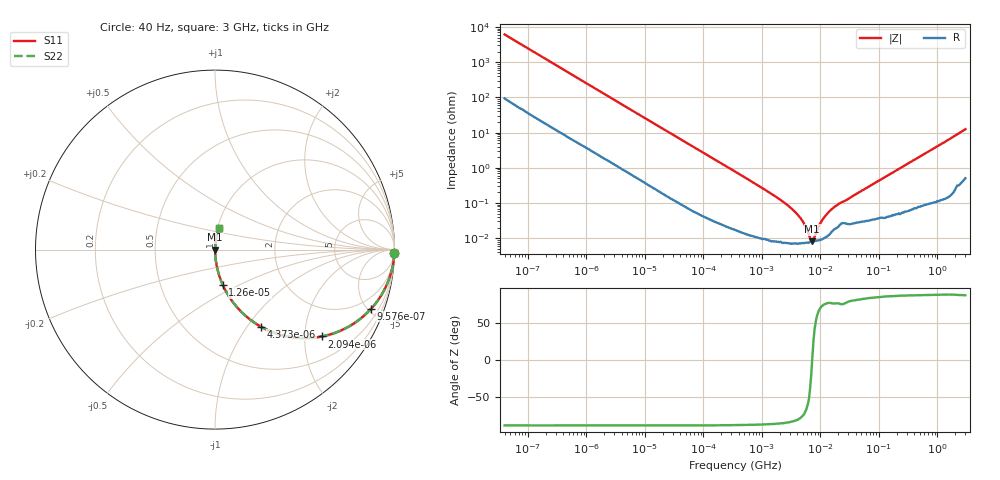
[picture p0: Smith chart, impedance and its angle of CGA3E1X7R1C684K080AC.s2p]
! S-parameter Generated by TDK Corporation
! Copyright(C) 2015 TDK Corporation.
! All Rights Reserved.
! TDK P/N: CGA3E1X7R1C684K080AC (Multilayer Ceramic Chip Capacitors)
! Property: C=680nF
! Size(LxWxT): 1.6x0.8x0.8mm, 0.063x0.031x0.031inches
! Model Type: s2p (Touchstone File Format Version 1.0)
! Frequency: DC=Yes Start=0.00004MHz Stop=3000MHz 396points Log-sweep
! Note: This model was converted from impedance.
! Model Generated on Jun. 23, 2015
! Hash(MD5):
! Port Assignments:
!  1 ---| |--- 2
! Applicable Conditions:
!  Temperature = 25 degC
!  DC Bias Voltage = 0 V
!  Small Signal Operation
! Terms and conditions regarding TDK Simulation Models
! (1)This simulation model is being provided solely for informational purposes. Please refer to the specifications of the products in terms of detailed characteristics of such products.
! (2)In no event shall TDK Corporation of any of its subsidiaries be liable for any loss or damage arising, directly or indirectly,
!  From any information contained in this simulation model, including, but not limited to loss or damages arising from any inaccuracies, omissions or errors in connection with such information.
! (3)Any and all copyrights on this simulation model are owned by TDK Corporation.
!  Duplication or redistribution of this simulation model without prior written permission from TDK Corporation is prohibited.
! (4)This simulation model is subject to any modification or change without any prior notice.
! (5)Neither TDK Corporation nor any of its subsidiaries shall make any warranty, express or implied,
!  Including but not limited to the correctness, implied warranties of merchantability and fitness for a particular purpose with respect to this simulation models.
! (6)The use of this simulation model shall be deemed to have consented to the terms and conditions hereof.
# MHz S MA R 50
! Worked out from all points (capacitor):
!   395 points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, 40 Hz to 3 GHz, reference 50 ohm
!   read as one part in series: C = 647 nF near 41.88 Hz
!   lowest |Z| = 8.17 mohm at 7.224 MHz (marker M1)
!   series resonance near 7.228 MHz, so ESL is about 750 pH
!   S11 on the Smith chart (normalised r, x): 40 Hz: open; 957.6 Hz: 1.08, -5.28; 2.094 kHz: 1.04, -2.43; 4.373 kHz: 1.02, -1.17; 12.6 kHz: 1.01, -0.41; 3 GHz: 1.01, +0.25
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4e-05  0.9996 -0.9  0.01629 88.2  0.01629 88.2  0.9996 -0.9
0.0002407527  0.994 -5.5  0.09569 83.7  0.09569 83.7  0.994 -5.5
0.000834128  0.9454 -18.2  0.3125 71.0  0.3125 71.0  0.9454 -18.2
0.0009576241  0.9306 -20.6  0.3527 68.5  0.3527 68.5  0.9306 -20.6
0.002094026  0.7664 -39.1  0.6313 50.0  0.6313 50.0  0.7664 -39.1
0.00437302  0.502 -59.0  0.8576 30.1  0.8576 30.1  0.502 -59.0
0.01260356  0.2011 -77.6  0.9767 11.6  0.9767 11.6  0.2011 -77.6
0.01739424  0.148 -80.7  0.9869 8.5  0.9869 8.5  0.148 -80.7
0.05496573  0.04836 -86.4  0.9981 2.8  0.9981 2.8  0.04836 -86.4
0.3464102  0.007855 -88.3  0.9998 0.4  0.9998 0.4  0.007855 -88.3
1.510739  0.001754 -87.2  0.9999 0.1  0.9999 0.1  0.001754 -87.2
3.154924  0.0007153 -84.3  0.9999 0.0  0.9999 0.0  0.0007153 -84.3
4.773931  0.000336 -77.4  0.9999 0.0  0.9999 0.0  0.000336 -77.4
5.480732  0.0002271 -70.8  0.9999 0.0  0.9999 0.0  0.0002271 -70.8
6.588528  0.0001055 -42.4  0.9999 0.0  0.9999 0.0  0.0001055 -42.4
7.22376  8.167e-05 -0.3  0.9999 0.0  0.9999 0.0  8.167e-05 -0.3
7.920238  0.0001096 40.9  0.9999 -0.0  0.9999 -0.0  0.0001096 40.9
9.092863  0.0001988 64.0  0.9999 -0.0  0.9999 -0.0  0.0001988 64.0
10.93076  0.0003444 73.9  0.9999 -0.0  0.9999 -0.0  0.0003444 73.9
15.79611  0.0006831 76.7  0.9998 -0.0  0.9998 -0.0  0.0006831 76.7
150.6385  0.006463 85.9  0.9996 -0.4  0.9996 -0.4  0.006463 85.9
3000  0.1233 80.6  0.9874 -7.1  0.9874 -7.1  0.1233 80.6
